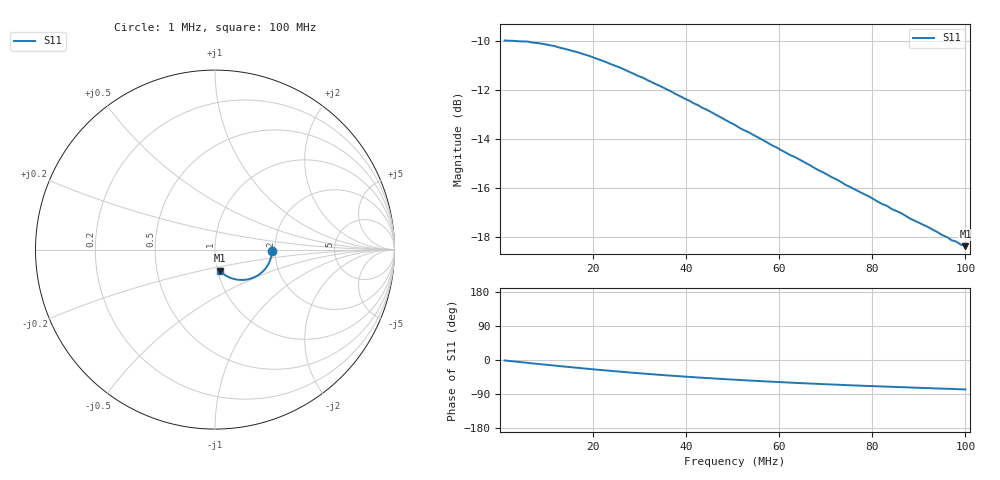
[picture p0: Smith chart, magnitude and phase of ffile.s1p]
# Hz S RI R 50.0
! written by SimSmith version 18.3c
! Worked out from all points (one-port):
!   101 points, 1 MHz to 100 MHz, reference 50 ohm
!   lowest |S11| = -18.4 dB at 100 MHz (marker M1), VSWR 1.27, Z = 51.2 - j12.2 ohm
!   |S11| at or under -10 dB: 3.642 MHz to end of sweep
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1000000  0.3171 -0.00695
5950000  0.313 -0.0412
1.09e7  0.3011 -0.0738
1.387e7  0.2913 -0.0907
1.684e7  0.2801 -0.1069
1.981e7  0.2675 -0.1208
2.575e7  0.2403 -0.1424
3.07e7  0.2162 -0.1557
3.565e7  0.1926 -0.1636
3.862e7  0.1789 -0.1665
4.456e7  0.154 -0.1692
5.05e7  0.1313 -0.1681
5.743e7  0.1079 -0.1641
6.337e7  0.0909 -0.1593
7.525e7  0.063 -0.1464
7.921e7  0.0559 -0.142
8.218e7  0.0506 -0.138
8.317e7  0.0492 -0.1372
8.416e7  0.0473 -0.1357
8.614e7  0.0443 -0.1339
8.812e7  0.0413 -0.131
9.208e7  0.036 -0.1269
9.505e7  0.0318 -0.123
9.604e7  0.0305 -0.1222
9.703e7  0.0295 -0.1205
9.802e7  0.028 -0.1201
9.901e7  0.0269 -0.1186
1e8  0.0257 -0.1179
